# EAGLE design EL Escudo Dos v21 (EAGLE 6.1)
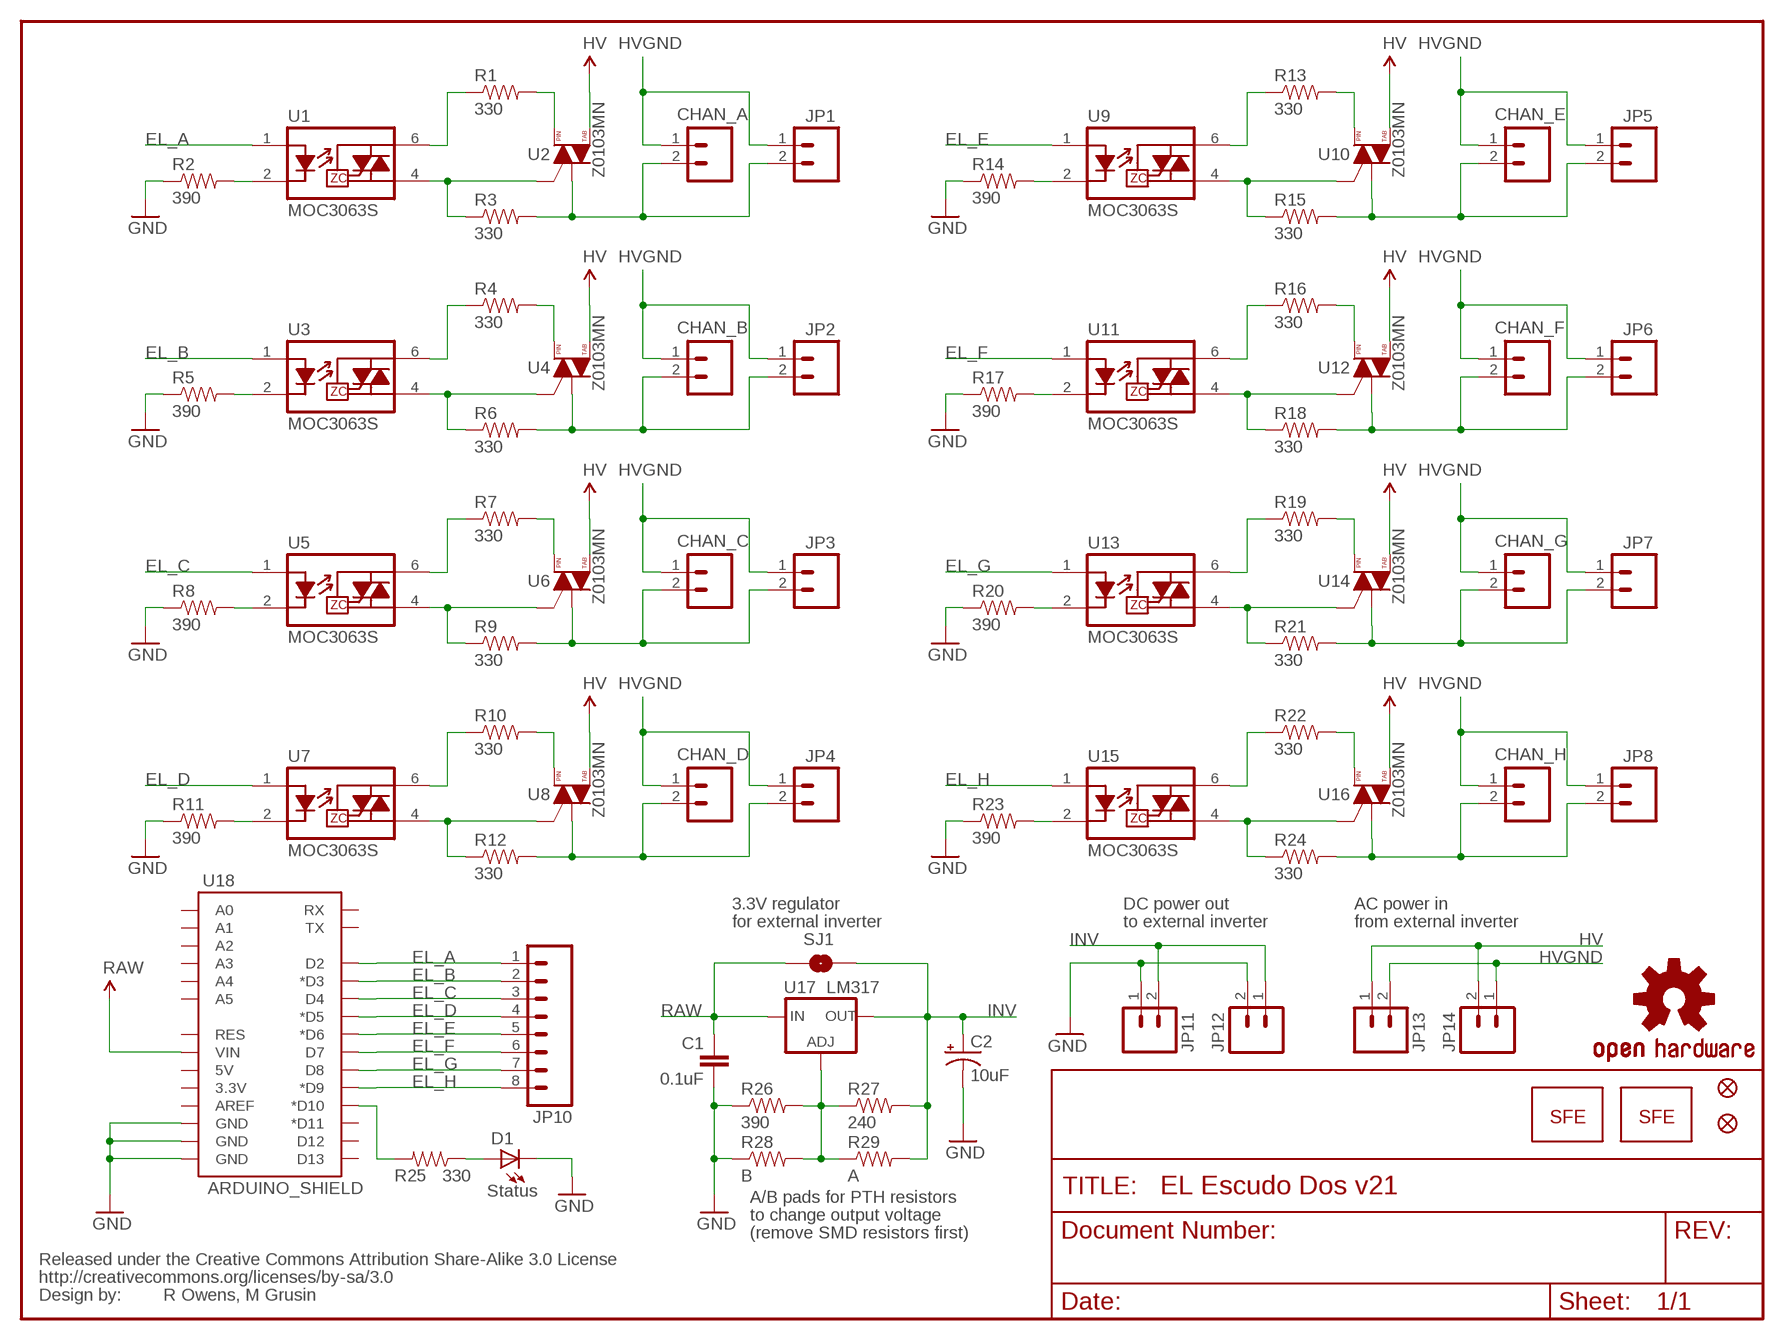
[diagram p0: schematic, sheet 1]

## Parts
C1  0.1uF  CAP0603-CAP  [0603-CAP]
C2  10uF  CAP_POL1206  [EIA3216]
CHAN_A  M02-JST-2MM-SMT  [JST-2-SMD]
CHAN_B  M02-JST-2MM-SMT  [JST-2-SMD]
CHAN_C  M02-JST-2MM-SMT  [JST-2-SMD]
CHAN_D  M02-JST-2MM-SMT  [JST-2-SMD]
CHAN_E  M02-JST-2MM-SMT  [JST-2-SMD]
CHAN_F  M02-JST-2MM-SMT  [JST-2-SMD]
CHAN_G  M02-JST-2MM-SMT  [JST-2-SMD]
CHAN_H  M02-JST-2MM-SMT  [JST-2-SMD]
D1  Status  LED0603  [LED-0603]
JP1  M02PTH  [1X02]
JP2  M02PTH  [1X02]
JP3  M02PTH  [1X02]
JP4  M02PTH  [1X02]
JP5  M02PTH  [1X02]
JP6  M02PTH  [1X02]
JP7  M02PTH  [1X02]
JP8  M02PTH  [1X02]
JP9  LOGO-SFENEW  [SFE-NEW-WEBLOGO]
JP10  M081X08  [1X08]
JP11  M02-JST-2MM-SMT  [JST-2-SMD]
JP12  M02PTH  [1X02]
JP13  M02PTH  [1X02]
JP14  M02-JST-2MM-SMT  [JST-2-SMD]
JP15  LOGO-SFENEW  [SFE-NEW-WEBLOGO]
JP16  FIDUCIALUFIDUCIAL  [MICRO-FIDUCIAL]
JP17  FIDUCIALUFIDUCIAL  [MICRO-FIDUCIAL]
R1  330  RESISTOR0603-RES  [0603-RES]
R2  390  RESISTOR0603-RES  [0603-RES]
R3  330  RESISTOR0603-RES  [0603-RES]
R4  330  RESISTOR0603-RES  [0603-RES]
R5  390  RESISTOR0603-RES  [0603-RES]
R6  330  RESISTOR0603-RES  [0603-RES]
R7  330  RESISTOR0603-RES  [0603-RES]
R8  390  RESISTOR0603-RES  [0603-RES]
R9  330  RESISTOR0603-RES  [0603-RES]
R10  330  RESISTOR0603-RES  [0603-RES]
R11  390  RESISTOR0603-RES  [0603-RES]
R12  330  RESISTOR0603-RES  [0603-RES]
R13  330  RESISTOR0603-RES  [0603-RES]
R14  390  RESISTOR0603-RES  [0603-RES]
R15  330  RESISTOR0603-RES  [0603-RES]
R16  330  RESISTOR0603-RES  [0603-RES]
R17  390  RESISTOR0603-RES  [0603-RES]
R18  330  RESISTOR0603-RES  [0603-RES]
R19  330  RESISTOR0603-RES  [0603-RES]
R20  390  RESISTOR0603-RES  [0603-RES]
R21  330  RESISTOR0603-RES  [0603-RES]
R22  330  RESISTOR0603-RES  [0603-RES]
R23  390  RESISTOR0603-RES  [0603-RES]
R24  330  RESISTOR0603-RES  [0603-RES]
R25  330  RESISTOR0603-RES  [0603-RES]
R26  390  RESISTOR0603-RES  [0603-RES]
R27  240  RESISTOR0603-RES  [0603-RES]
R28  B  RESISTORPTH-1/4W  [AXIAL-0.4]
R29  A  RESISTORPTH-1/4W  [AXIAL-0.4]
SJ1  SOLDERJUMPERNO  [SJ_2S-NO]
U1  MOC3063S  [DIP8SMD]
U2  Z0103MN  TRIACSMD  [SOT223]
U3  MOC3063S  [DIP8SMD]
U4  Z0103MN  TRIACSMD  [SOT223]
U5  MOC3063S  [DIP8SMD]
U6  Z0103MN  TRIACSMD  [SOT223]
U7  MOC3063S  [DIP8SMD]
U8  Z0103MN  TRIACSMD  [SOT223]
U9  MOC3063S  [DIP8SMD]
U10  Z0103MN  TRIACSMD  [SOT223]
U11  MOC3063S  [DIP8SMD]
U12  Z0103MN  TRIACSMD  [SOT223]
U13  MOC3063S  [DIP8SMD]
U14  Z0103MN  TRIACSMD  [SOT223]
U15  MOC3063S  [DIP8SMD]
U16  Z0103MN  TRIACSMD  [SOT223]
U17  LM317  V_REG_317DPACK  [V-REG_DPACK]
U18  ARDUINO_SHIELD  ARDUINO_SHIELDNOLABELS  [DUEMILANOVE_SHIELD_NOLABELS]
U$4  CREATIVE_COMMONS  [CREATIVE_COMMONS]
U$5  OSHW-LOGOS  [OSHW-LOGO-S]

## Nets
EL_A: JP10.1 U1.1(A) U18.D2
EL_B: JP10.2 U3.1(A) U18.D3(*D3)
EL_C: JP10.3 U5.1(A) U18.D4
EL_D: JP10.4 U7.1(A) U18.D5(*D5)
EL_E: JP10.5 U9.1(A) U18.D6(*D6)
EL_F: JP10.6 U11.1(A) U18.D7
EL_G: JP10.7 U13.1(A) U18.D8
EL_H: JP10.8 U15.1(A) U18.D9(*D9)
GND: C1.2 C2.C(-) D1.C JP11.1 JP12.2 R2.1 R5.1 R8.1 R11.1 R14.1 R17.1 R20.1 R23.1 R26.1 R28.P$1 U18.GND@0(GND) U18.GND@1(GND) U18.GND@2(GND)
HV: JP13.1 JP14.2 U2.4(T2) U4.4(T2) U6.4(T2) U8.4(T2) U10.4(T2) U12.4(T2) U14.4(T2) U16.4(T2)
HVGND: CHAN_A.1 CHAN_B.1 CHAN_C.1 CHAN_D.1 CHAN_E.1 CHAN_F.1 CHAN_G.1 CHAN_H.1 JP1.1 JP2.1 JP3.1 JP4.1 JP5.1 JP6.1 JP7.1 JP8.1 JP13.2 JP14.1
INV: C2.A(+) JP11.2 JP12.1 R27.2 R29.P$2 SJ1.2 U17.4(OUT)
N$1: R2.2 U1.2(K)
N$2: R26.2 R27.1 R28.P$2 R29.P$1 U17.1(ADJ)
N$3: R1.1 U1.6(T1)
N$4: R25.2 U18.D10(*D10)
N$5: R6.1 U3.4(T2) U4.3(G)
N$6: R5.2 U3.2(K)
N$7: R4.1 U3.6(T1)
N$8: CHAN_B.2 JP2.2 R6.2 U4.1(T1)
N$9: R1.2 U2.2(T2)
N$10: R9.1 U5.4(T2) U6.3(G)
N$11: R8.2 U5.2(K)
N$12: R7.1 U5.6(T1)
N$13: CHAN_C.2 JP3.2 R9.2 U6.1(T1)
N$14: D1.A R25.1
N$15: R4.2 U4.2(T2)
N$16: R12.1 U7.4(T2) U8.3(G)
N$17: R11.2 U7.2(K)
N$18: R10.1 U7.6(T1)
N$19: CHAN_D.2 JP4.2 R12.2 U8.1(T1)
N$20: R7.2 U6.2(T2)
N$21: CHAN_A.2 JP1.2 R3.2 U2.1(T1)
N$22: R15.1 U9.4(T2) U10.3(G)
N$23: R14.2 U9.2(K)
N$24: R13.1 U9.6(T1)
N$25: CHAN_E.2 JP5.2 R15.2 U10.1(T1)
N$26: R10.2 U8.2(T2)
N$27: R18.1 U11.4(T2) U12.3(G)
N$28: R17.2 U11.2(K)
N$29: R16.1 U11.6(T1)
N$30: CHAN_F.2 JP6.2 R18.2 U12.1(T1)
N$31: R13.2 U10.2(T2)
N$32: R21.1 U13.4(T2) U14.3(G)
N$33: R20.2 U13.2(K)
N$34: R19.1 U13.6(T1)
N$35: CHAN_G.2 JP7.2 R21.2 U14.1(T1)
N$36: R16.2 U12.2(T2)
N$37: R24.1 U15.4(T2) U16.3(G)
N$38: R23.2 U15.2(K)
N$39: R22.1 U15.6(T1)
N$40: CHAN_H.2 JP8.2 R24.2 U16.1(T1)
N$41: R19.2 U14.2(T2)
N$42: R22.2 U16.2(T2)
N$117: R3.1 U1.4(T2) U2.3(G)
RAW: C1.1 SJ1.1 U17.3(IN) U18.VIN
Unconnected: U18.3.3V U18.5V U18.A0 U18.A1 U18.A2 U18.A3 U18.A4 U18.A5 U18.AREF U18.D11(*D11) U18.D12 U18.D13 U18.RES U18.RX U18.TX

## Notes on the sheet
- 3.3V regulator | DC power out | AC power in
- for external inverter | to external inverter | from external inverter
- A/B pads for PTH resistors
- to change output voltage
- (remove SMD resistors first)
- R Owens, M Grusin

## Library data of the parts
C1 = SparkFun:CAP: Capacitor
C2 = SparkFun:CAP_POL: Capacitor Polarized
CHAN_A CHAN_B CHAN_C CHAN_D CHAN_E CHAN_F CHAN_G CHAN_H JP1-JP8 JP11-JP14 = SparkFun:M02: Header 2
D1 = SparkFun:LED: LEDs
JP9 JP15 = SparkFun:LOGO-SFE: Spark Fun Electronics PCB Logo
JP10 = SparkFun:M08: Header 8 Standard 8-pin 0.1" header. Use with straight break away headers (SKU : PRT-00116), right angle break away headers (PRT-00553), swiss pins (PRT-00743), machine pins (PRT-00117), and female headers (PRT-00115).
JP16 JP17 = SparkFun:FIDUCIAL: Fiducial Alignment Points
R1-R29 = SparkFun:RESISTOR: Resistor
SJ1 = SparkFun:SOLDERJUMPER: Solder Jumper
U1 U3 U5 U7 U9 U11 U13 U15 = mike-temp:MOC3063*: Optotriac in DIP and SMD LED: Vf: 1.2V If: 5 mA TRIAC Vdrm: 600V Itsm: 1A Viso: 5000V DV/dt: 1500V/us DIP: MOC3063 SMD: MOC3063S
U2 U4 U6 U8 U10 U12 U14 U16 = mike-temp:TRIAC
U17 = SparkFun:V_REG_317: Voltage Regulator Standard LM317 adjustable voltage regulator. AOI (Adjust Output Input). Google 'LM317 Calculator' for easy to use app to get the two resistor values needed. 240/720 for 5V output. 240/390 for 3.3V output. Spark Fun Electronics SKU : COM-00527
U18 = SparkFun:ARDUINO_SHIELD
U$4 = SparkFun:CREATIVE_COMMONS
U$5 = SparkFun:OSHW-LOGO: Open Source Hardware Logo This logo indicates the piece of hardware it is found on incorporates a OSHW license and/or adheres to the definition of open source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

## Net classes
0 Default: width 0.203 mm
1 VCC: width 0.305 mm
2 GND: width 0.813 mm
3 HV: width 0.381 mm

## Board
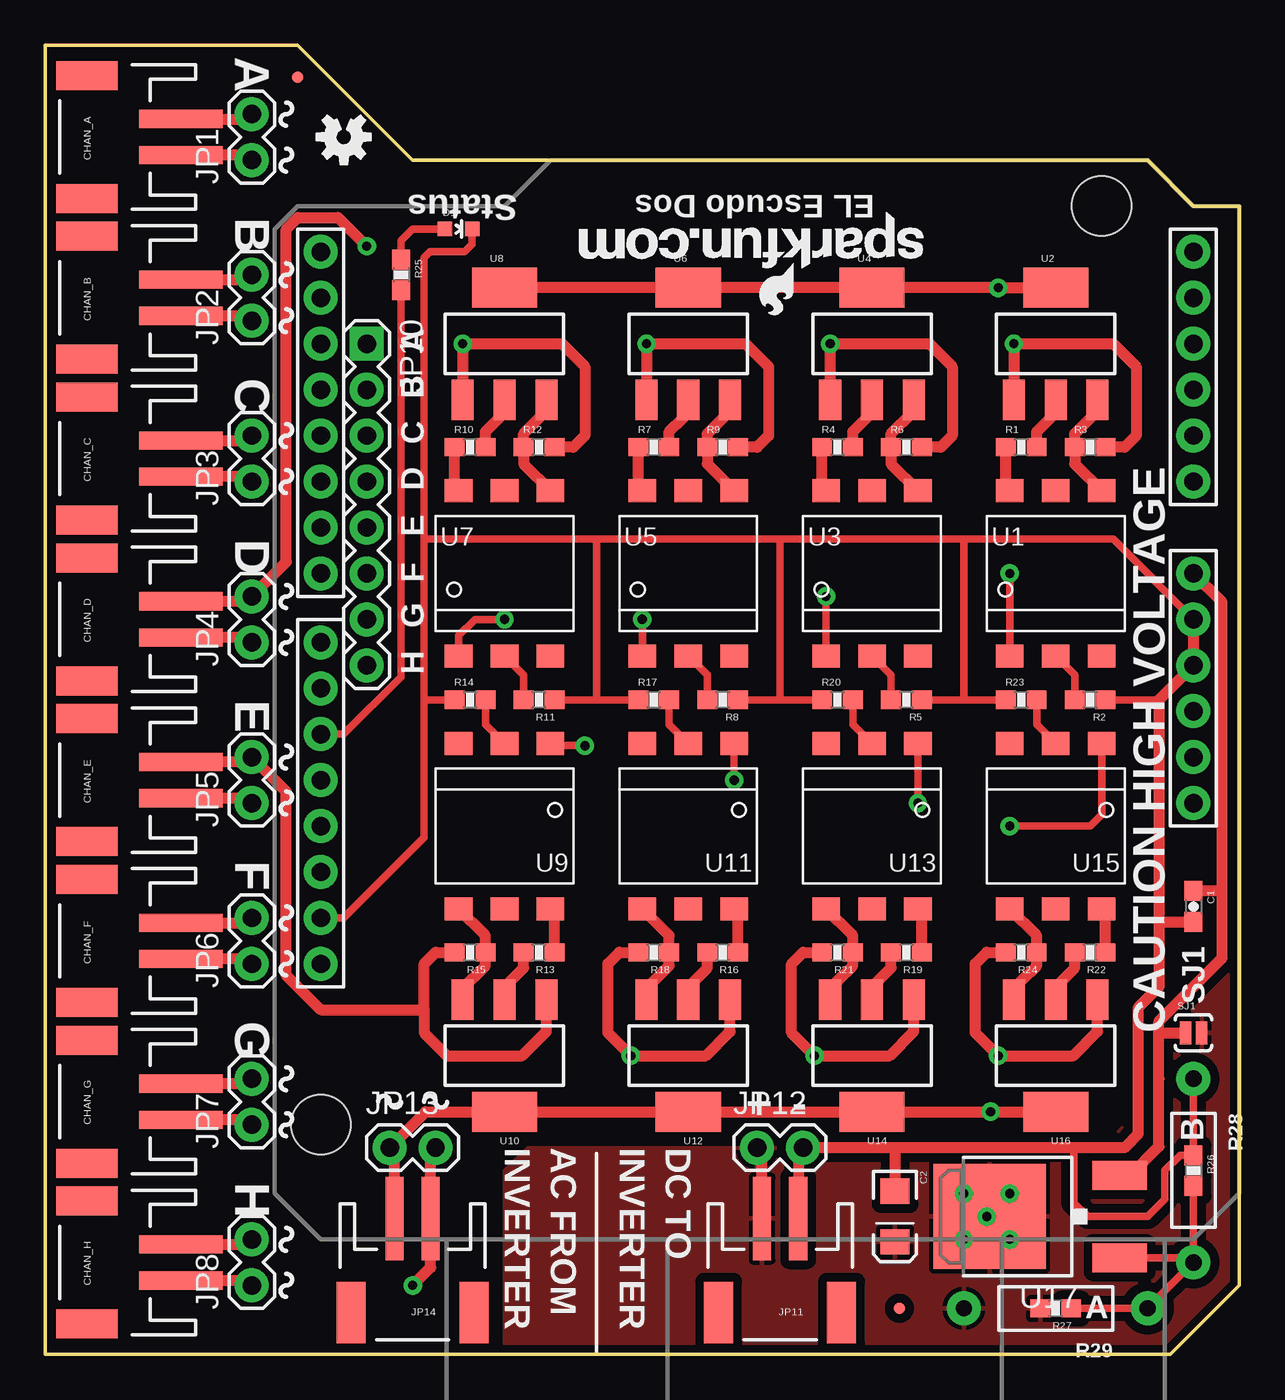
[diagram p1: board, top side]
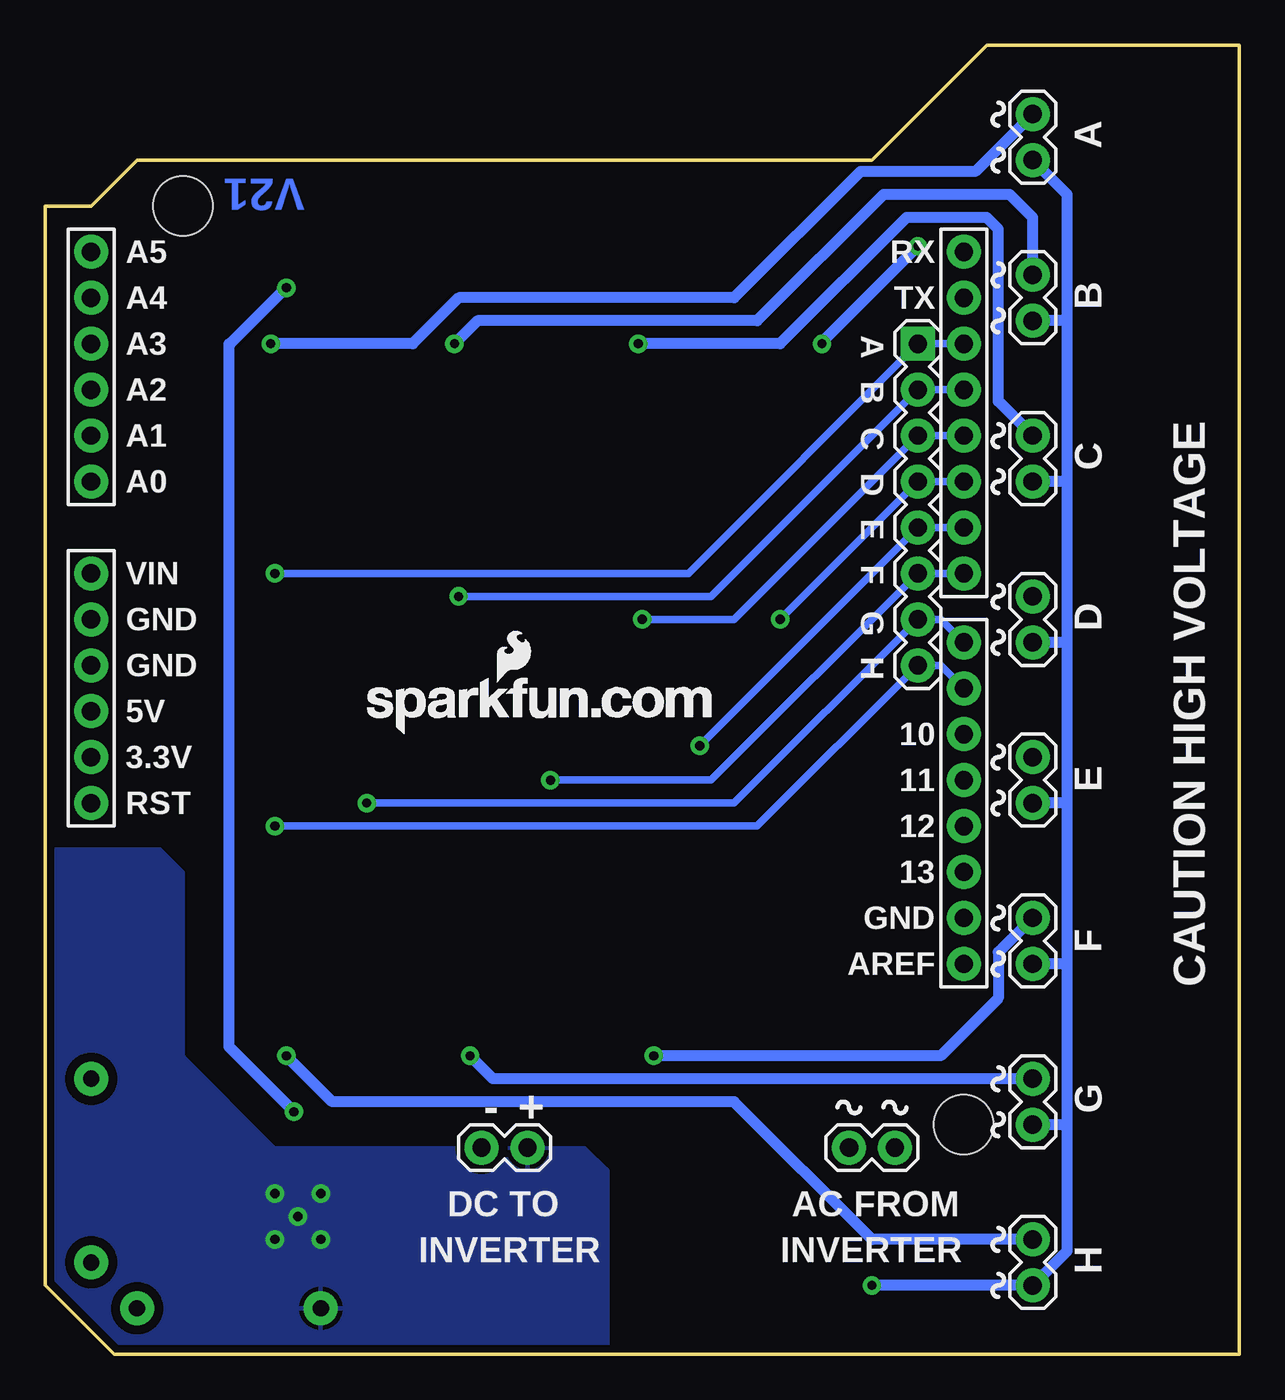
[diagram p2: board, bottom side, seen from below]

Size 66.04 x 72.39 mm. Coordinates in mm from the lower left corner, seen from the top.
Outline: 20.32,66.04 13.97,72.39 0,72.39 0,0 62.23,0 66.04,3.81 66.04,63.5 63.5,63.5 60.96,66.04 20.32,66.04
Copper layers (1*16): Top 0.035mm / dielectric 1.5mm / Bottom 0.035mm
Design rules: minimum track width 8mil, minimum drill 20mil, track to track 0.5mm, track to pad 0.5mm, pad to pad 0.5mm, via to via 0.5mm, smd to smd 8mil, copper to edge 10mil, drill to drill 8mil, minimum pad ring 12mil, minimum via ring 10mil, stop-mask expansion 4mil, vias tented up to drill 25mil, thermal gap 10mil

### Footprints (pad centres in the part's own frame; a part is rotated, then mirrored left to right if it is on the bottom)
0603-CAP = smd 1.1 x 1: 1 -0.85,0; 2 0.85,0
EIA3216 = smd 1.4 x 1.6: A 1.4,0; C -1.4,0
JST-2-SMD = smd 1 x 4.6: 1 -1,-3.7; 2 1,-3.7 | smd 1.6 x 3.4: NC1 -3.4,1.5; NC2 3.4,1.5
LED-0603 = smd 0.8 x 0.8: A 0,-0.75; C 0,0.75
1X02 = drill 1.016 pad 1.88: 1 0,0; 2 2.54,0
1X08 = drill 1.016 pad 1.88 square: 1 0,0 | drill 1.016 pad 1.88: 2 2.54,0; 3 5.08,0; 4 7.62,0; 5 10.16,0; 6 12.7,0; 7 15.24,0; 8 17.78,0
MICRO-FIDUCIAL = smd 0.635 x 0.635: 1 0,0
0603-RES = smd 1.1 x 1: 1 -0.85,0; 2 0.85,0
AXIAL-0.4 = drill 0.9 pad 1.88: P$1 -5.08,0; P$2 5.08,0
SJ_2S-NO = smd 0.635 x 1.27: 1 -0.45,0; 2 0.45,0
DIP8SMD = smd 1.524 x 1.27: 1 -2.54,-4.572; 2 0,-4.572; 3 2.54,-4.572; 4 2.54,4.572; 5 0,4.572; 6 -2.54,4.572
SOT223 = smd 1.219 x 2.235: 1 -2.311,-3.099; 2 0,-3.099; 3 2.311,-3.099 | smd 3.6 x 2.2: 4 0,3.099
V-REG_DPACK = smd 1.6 x 3: 1 -2.28,-4.8; 3 2.28,-4.8 | smd 5.8 x 6.2: 4 0,2.38
DUEMILANOVE_SHIELD_NOLABELS = drill 1.016 pad 1.88: 3.3V 50.8,26.67; 5V 50.8,29.21; A0 50.8,41.91; A1 50.8,44.45; A2 50.8,46.99; A3 50.8,49.53; A4 50.8,52.07; A5 50.8,54.61; AREF 2.54,15.24; D2 2.54,49.53; D3 2.54,46.99; D4 2.54,44.45; D5 2.54,41.91; D6 2.54,39.37; D7 2.54,36.83; D8 2.54,33.02; D9 2.54,30.48; D10 2.54,27.94; D11 2.54,25.4; D12 2.54,22.86; D13 2.54,20.32; GND@0 50.8,31.75; GND@1 50.8,34.29; GND@2 2.54,17.78; RES 50.8,24.13; RX 2.54,54.61; TX 2.54,52.07; VIN 50.8,36.83 | hole 3.302: 45.72,57.15; 2.54,6.35

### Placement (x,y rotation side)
C1  63.5,24.77 270 top
C2  46.99,7.62 270 top
CHAN_A  3.81,67.31 90 top
CHAN_B  3.81,58.42 90 top
CHAN_C  3.81,49.53 90 top
CHAN_D  3.81,40.64 90 top
CHAN_E  3.81,31.75 90 top
CHAN_F  3.81,22.86 90 top
CHAN_G  3.81,13.97 90 top
CHAN_H  3.81,5.08 90 top
D1  22.86,62.23 270 top
JP1  11.43,66.04 90 top
JP2  11.43,57.15 90 top
JP3  11.43,48.26 90 top
JP4  11.43,39.37 90 top
JP5  11.43,30.48 90 top
JP6  11.43,21.59 90 top
JP7  11.43,12.7 90 top
JP8  11.43,3.81 90 top
JP9  48.58,63.18 180 top
JP10  17.78,55.88 270 top
JP11  40.64,3.81 180 top
JP12  39.37,11.43 0 top
JP13  19.05,11.43 0 top
JP14  20.32,3.81 180 top
JP15  48.26,34.29 0 bottom
JP16  13.97,70.61 0 top
JP17  47.24,2.54 0 top
R1  53.98,50.16 0 top
R2  57.78,36.2 180 top
R3  57.78,50.16 0 top
R4  43.81,50.16 0 top
R5  47.62,36.2 180 top
R6  47.62,50.16 0 top
R7  33.66,50.16 0 top
R8  37.47,36.2 180 top
R9  37.47,50.16 0 top
R10  23.5,50.16 0 top
R11  27.3,36.2 180 top
R12  27.3,50.16 0 top
R13  27.3,22.23 180 top
R14  23.5,36.2 0 top
R15  23.5,22.23 180 top
R16  37.47,22.23 180 top
R17  33.66,36.2 0 top
R18  33.66,22.23 180 top
R19  47.62,22.23 180 top
R20  43.81,36.2 0 top
R21  43.81,22.23 180 top
R22  57.78,22.23 180 top
R23  53.98,36.2 0 top
R24  53.98,22.23 180 top
R25  19.68,59.69 270 top
R26  63.5,10.16 270 top
R27  55.88,2.54 180 top
R28  63.5,10.16 270 top
R29  55.88,2.54 180 top
SJ1  63.5,17.78 0 top
U1  55.88,43.18 0 top
U2  55.88,55.88 0 top
U3  45.72,43.18 0 top
U4  45.72,55.88 0 top
U5  35.56,43.18 0 top
U6  35.56,55.88 0 top
U7  25.4,43.18 0 top
U8  25.4,55.88 0 top
U9  25.4,29.21 180 top
U10  25.4,16.51 180 top
U11  35.56,29.21 180 top
U12  35.56,16.51 180 top
U13  45.72,29.21 180 top
U14  45.72,16.51 180 top
U15  55.88,29.21 180 top
U16  55.88,16.51 180 top
U17  54.61,7.62 90 top
U18  12.7,6.35 0 top
U$4  not placed on the board
U$5  16.51,67.31 180 top

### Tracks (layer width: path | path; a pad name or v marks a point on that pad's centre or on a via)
EL_A  (via drill 0.51)
  Top 0.406: v53.34,43.18 U1.1
  Bottom 0.406: v53.34,43.18 30.48,43.18 JP10.1 U18.D2
EL_B  (via drill 0.51)
  Top 0.406: v43.18,41.91 U3.1
  Bottom 0.406: v43.18,41.91 29.21,41.91 JP10.2 U18.D3
EL_C  (via drill 0.51)
  Top 0.406: v33.02,40.64 U5.1
  Bottom 0.406: v33.02,40.64 27.94,40.64 JP10.3 U18.D4
EL_D  (via drill 0.51)
  Top 0.406: U7.1 22.86,39.74 23.76,40.64 v25.4,40.64
  Bottom 0.406: v25.4,40.64 JP10.4 U18.D5
EL_E  (via drill 0.51)
  Top 0.406: v29.84,33.66 27.94,33.66 U9.1
  Bottom 0.406: v29.84,33.66 JP10.5 U18.D6
EL_F  (via drill 0.51)
  Top 0.406: v38.1,31.75 U11.1
  Bottom 0.406: v38.1,31.75 29.21,31.75 JP10.6 U18.D7
EL_G  (via drill 0.51)
  Top 0.406: v48.26,30.48 U13.1
  Bottom 0.406: v48.26,30.48 27.94,30.48 JP10.7 16.51,40.64 U18.D8
EL_H  (via drill 0.51)
  Top 0.406: v53.34,29.21 57.78,29.21 58.42,29.84 U15.1
  Bottom 0.406: v53.34,29.21 26.67,29.21 JP10.8 16.51,38.1 U18.D9
GND
  Top 0.406: 20.95,45.09 30.48,45.09 | 30.48,45.09 40.64,45.09 | 40.64,45.09 50.8,45.09 | 50.8,36.2 R23.1 | 50.8,45.09 50.8,36.2 | 40.64,36.2 R20.1 | 40.64,45.09 40.64,36.2 | 30.48,36.2 R17.1 | 30.48,45.09 30.48,36.2 | 30.48,36.2 R11.1 | 40.64,36.2 R8.1 | 50.8,36.2 R5.1 | 20.95,36.2 R14.1 | 20.95,36.2 20.95,45.09 | 50.8,45.09 59.05,45.09 U18.GND@1 | 56.9,11.43 56.9,8.38 57.66,7.62 60.96,7.62 61.91,8.57 61.91,10.16 62.76,11.01 R26.1 R28.P$1 | 61.59,36.2 R2.1 | D1.C 23.61,61.39 23.18,60.96 21.27,60.96 20.95,60.64 20.95,45.09 | 20.95,36.2 20.95,28.57 16.51,24.13 U18.GND@2
  Top 0.61: JP11.1 41.64,11.16 JP12.2 46.99,11.43 | 46.99,11.43 C2.C | 46.99,11.43 56.9,11.43 59.69,11.43 60.43,12.17 60.43,19.15 61.59,20.32 61.59,23.91 | U18.GND@1 U18.GND@0 61.59,36.2 61.59,23.91 | 61.59,23.91 C1.2
HV  (via drill 0.51)
  Top 0.61: JP14.2 19.32,11.16 JP13.1 21.03,13.41 U10.4 U12.4 U14.4 v52.29,13.41 U16.4 | U8.4 U6.4 U4.4 v52.7,58.98 U2.4
  Bottom 0.61: v52.29,13.41 55.88,17 55.88,55.88 55.8,55.88 v52.7,58.98
HVGND  (via drill 0.51)
  Top 0.61: JP1.1 11.16,66.31 CHAN_A.1 | JP2.1 11.16,57.42 CHAN_B.1 | JP3.1 11.16,48.53 CHAN_C.1 | JP4.1 11.16,39.64 CHAN_D.1 | JP5.1 11.16,30.75 CHAN_E.1 | JP6.1 11.16,21.86 CHAN_F.1 | JP7.1 11.16,12.97 CHAN_G.1 | JP8.1 11.16,4.08 CHAN_H.1 | v20.32,3.81 21.32,4.81 JP14.1 21.32,11.16 JP13.2
  Bottom 0.61: JP1.1 9.53,64.14 9.53,57.15 | 9.53,57.15 JP2.1 | 9.53,48.26 9.53,57.15 | 9.53,48.26 JP3.1 | 9.53,39.37 9.53,48.26 | 9.53,39.37 JP4.1 | 9.53,30.48 9.53,39.37 | 9.53,30.48 JP5.1 | 9.53,21.59 9.53,30.48 | 9.53,21.59 JP6.1 | 9.53,12.7 9.53,21.59 | 9.53,12.7 JP7.1 | 9.53,12.7 9.53,5.71 JP8.1 v20.32,3.81
INV  (via drill 0.51)
  Top 0.61: JP11.2 39.64,11.16 JP12.1
  other vias: 50.8,6.35 50.8,8.89 53.34,8.89 53.34,6.35 52.07,7.62
  pour Bottom (isolate 0.406): 34.92,0 34.92,10.16 36.2,11.43 53.34,11.43 58.42,16.51 58.42,26.67 59.69,27.94 66.04,27.94 66.04,3.81 62.23,0
  pour Top (isolate 0.406): 62.23,0 25.4,0 25.4,10.16 26.67,11.43 58.42,11.43 60.96,13.97 60.96,17.78 66.04,22.86 66.04,3.81
N$1
  Top 0.406: R2.2 56.94,37.55 U1.2
N$2
  Top 0.406: R27.1 R29.P$1 62.23,3.81 R28.P$2 R26.2 | 63.24,5.34 U17.1
  Top 0.61: R28.P$2 63.24,5.34
N$3
  Top 0.61: R1.1 53.12,47.97 U1.6
N$4
  Top 0.406: R25.2 19.68,37.47 16.51,34.29 U18.D10
N$5
  Top 0.61: U3.4 46.77,49.24 R6.1 46.77,50.9 47.94,52.07 47.94,52.69 U4.3
N$6
  Top 0.406: R5.2 46.77,37.55 U3.2
N$7
  Top 0.61: R4.1 42.97,47.97 U3.6
N$8  (via drill 0.51)
  Top 0.61: JP2.2 11.16,59.42 CHAN_B.2 | R6.2 49.53,50.16 50.16,50.8 50.16,54.61 48.9,55.88 v43.41,55.88 U4.1
  Bottom 0.61: JP2.2 11.43,62.87 12.7,64.14 19.68,64.14 26.67,57.15 42.14,57.15 v43.41,55.88
N$9
  Top 0.61: R1.2 54.83,51.02 55.88,52.07 U2.2
N$10
  Top 0.61: U5.4 36.62,49.24 R9.1 36.62,50.9 37.78,52.07 37.78,52.69 U6.3
N$11
  Top 0.406: R8.2 36.62,37.55 U5.2
N$12
  Top 0.61: R7.1 32.8,47.97 U5.6
N$13  (via drill 0.51)
  Top 0.61: JP3.2 11.16,50.53 CHAN_C.2 | R9.2 39.37,50.16 40.01,50.8 40.01,54.61 38.73,55.88 v33.25,55.88 U6.1
  Bottom 0.61: JP3.2 13.34,52.7 13.34,62.23 13.97,62.87 18.41,62.87 25.4,55.88 v33.25,55.88
N$14
  Top 0.406: R25.1 19.68,61.59 20.32,62.23 D1.A
N$15
  Top 0.61: R4.2 44.66,51.02 45.72,52.07 U4.2
N$16
  Top 0.61: U7.4 26.45,49.24 R12.1 26.45,50.9 27.62,52.07 27.71,52.16 U8.3
N$17
  Top 0.406: R11.2 26.45,37.55 U7.2
N$18
  Top 0.61: R10.1 22.64,47.97 U7.6
N$19  (via drill 0.51)
  Top 0.61: CHAN_D.2 11.16,41.64 JP4.2 13.34,43.81 13.34,62.23 13.97,62.87 16.19,62.87 v17.78,61.28 | R12.2 29.21,50.16 29.84,50.8 29.84,54.61 28.57,55.88 v23.09,55.88 U8.1
  Bottom 0.61: v23.09,55.88 23.09,55.97 v17.78,61.28
N$20
  Top 0.61: R7.2 34.51,51.02 35.24,51.75 35.56,52.07 U6.2
N$21  (via drill 0.51)
  Top 0.61: JP1.2 11.16,68.31 CHAN_A.2 | R3.2 59.69,50.16 60.33,50.8 60.33,54.61 59.05,55.88 v53.57,55.88 U2.1
  Bottom 0.61: JP1.2 14.61,65.41 20.95,65.41 27.94,58.42 43.18,58.42 45.72,55.88 v53.57,55.88
N$22
  Top 0.61: U9.4 24.34,23.15 R15.1 24.34,21.49 23.09,20.23 U10.3
N$23
  Top 0.406: R14.2 24.34,34.84 U9.2
N$24
  Top 0.61: R13.1 28.16,24.42 U9.6
N$25
  Top 0.61: CHAN_E.2 11.16,32.75 JP5.2 13.34,31.11 13.34,20.95 15.24,19.05 20.95,19.05 | 20.95,19.05 20.95,17.78 22.23,16.51 26.38,16.51 27.71,17.84 U10.1 | 20.95,19.05 20.95,21.59 21.59,22.23 R15.2
N$26
  Top 0.61: R10.2 24.34,51.02 25.4,52.07 U8.2
N$27
  Top 0.61: U11.4 34.51,23.15 R18.1 34.51,21.49 33.66,20.64 33.25,20.23 U12.3
N$28
  Top 0.406: R17.2 34.51,34.84 U11.2
N$29
  Top 0.61: R16.1 38.31,24.42 U11.6
N$30  (via drill 0.51)
  Top 0.61: JP6.2 11.16,23.86 CHAN_F.2 | R18.2 31.75,22.23 31.11,21.59 31.11,17.78 v32.38,16.51 36.54,16.51 37.87,17.84 U12.1
  Bottom 0.61: JP6.2 13.34,22.23 13.34,19.68 16.51,16.51 v32.38,16.51
N$31
  Top 0.61: R13.2 26.45,21.38 25.4,20.32 U10.2
N$32
  Top 0.61: U13.4 44.66,23.15 R21.1 44.66,21.49 43.81,20.64 43.41,20.23 U14.3
N$33
  Top 0.406: R20.2 44.66,34.84 U13.2
N$34
  Top 0.61: R19.1 48.48,24.42 U13.6
N$35  (via drill 0.51)
  Top 0.61: JP7.2 11.16,14.97 CHAN_G.2 | R21.2 41.91,22.23 41.27,21.59 41.27,17.78 v42.55,16.51 46.7,16.51 48.03,17.84 U14.1
  Bottom 0.61: JP7.2 41.27,15.24 v42.55,16.51
N$36
  Top 0.61: R16.2 36.62,21.38 35.56,20.32 U12.2
N$37
  Top 0.61: U15.4 54.83,23.15 R24.1 54.83,21.49 53.98,20.64 53.57,20.23 U16.3
N$38
  Top 0.406: R23.2 54.83,34.84 U15.2
N$39
  Top 0.61: R22.1 58.63,24.42 U15.6
N$40  (via drill 0.51)
  Top 0.61: JP8.2 11.16,6.08 CHAN_H.2 | R24.2 52.07,22.23 51.44,21.59 51.44,17.78 v52.7,16.51 56.86,16.51 58.19,17.84 U16.1
  Bottom 0.61: JP8.2 20.32,6.35 27.94,13.97 50.16,13.97 v52.7,16.51
N$41
  Top 0.61: R19.2 46.77,21.38 45.72,20.32 U14.2
N$42
  Top 0.61: R22.2 56.94,21.38 55.88,20.32 U16.2
N$117
  Top 0.61: U2.3 58.19,52.16 56.94,50.9 R3.1 56.94,49.24 U1.4
RAW
  Top 0.61: U17.3 60.01,9.9 | 60.01,9.9 60.54,9.9 | U18.VIN 65.09,41.59 65.09,25.61 | 61.59,17.78 61.59,15.24 61.59,11.49 60.01,9.9 | 61.59,17.78 61.59,18.41 65.09,21.91 65.09,25.61 | 65.09,25.61 C1.1 | 61.59,17.78 SJ1.1

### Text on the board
Bottom: V21
tPlace: A | Status | EL Escudo Dos | B | A | C | B | C | D | D | E | F | G | H | E | F | SJ1 | G | CAUTION HIGH VOLTAGE | + | - | INVERTER | AC FROM | INVERTER | DC TO | H
bPlace: A | RX | A5 | TX | B | A4 | A | A3 | B | A2 | C | A1 | C | D | A0 | E | F | VIN | G | D | GND | H | GND | 10 | 5V | 11 | 3.3V | E | 12 | RST | 13 | GND | F | AREF | CAUTION HIGH VOLTAGE | + | - | G | AC FROM | DC TO | INVERTER | INVERTER | H
tValues: R Owens, M Grusin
